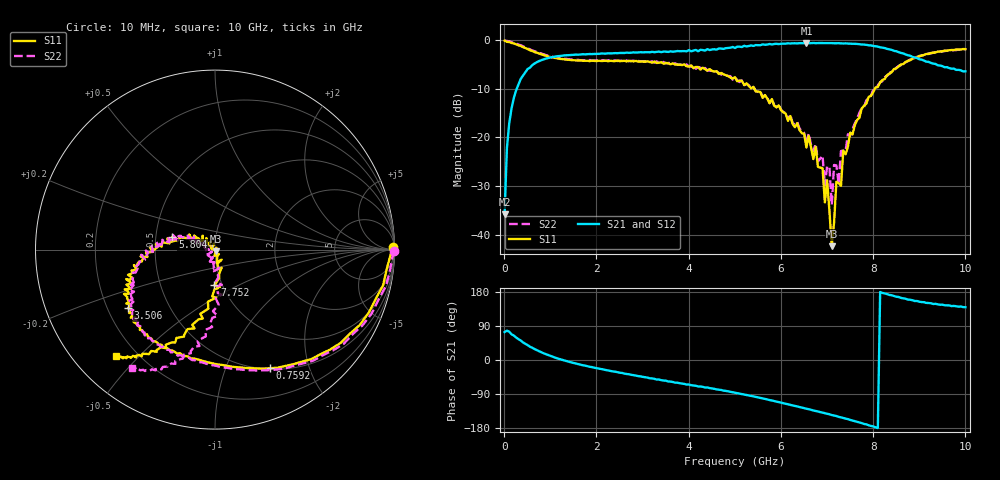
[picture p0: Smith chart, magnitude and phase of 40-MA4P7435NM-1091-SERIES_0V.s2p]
!Agilent Technologies,E8364C,MY48140145,A.09.42.15
!Agilent E8364C: A.09.42.15
!Date: Wednesday, December 02, 2020 13:39:51
!Correction: S11(Full 2 Port(1,2))
!S21(Full 2 Port(1,2))
!S12(Full 2 Port(1,2))
!S22(Full 2 Port(1,2))
!S2P File: Measurements: S11, S21, S12, S22:
# Hz S  dB  R 50
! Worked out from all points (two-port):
!   201 points, 10 MHz to 10 GHz, reference 50 ohm
!   highest |S21| = -0.57 dB at 6.553 GHz (marker M1); lowest = -35.8 dB at 10 MHz (marker M2)
!   |S21| within 3 dB of the highest: 994.4 MHz to 8.913 GHz (7.918 GHz wide, 160 % of centre)
!   lowest |S11| = -42.3 dB at 7.103 GHz (marker M3), VSWR 1.02, Z = 50.3 - j0.713 ohm
!   |S11| at or under -10 dB: 5.427 GHz to 8.037 GHz (2.611 GHz wide, 38.8 % of centre)
!   |S22| runs from -33.9 to 0.0 dB; largest |S21 - S12| = 0.023
!   S11 on the Smith chart (normalised r, x): 10 MHz: open; 759.2 MHz: 0.51, -1.44; 3.506 GHz: 0.29, -0.28; 5.804 GHz: 0.61, +0.09; 7.752 GHz: 0.92, -0.38; 10 GHz: 0.12, -0.43
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1e7  -0.10 0.7  -35.76 73.6  -37.67 50.6  -0.05 -0.4
5.995e7  -0.33 -6.7  -22.20 77.4  -22.18 78.0  -0.16 -6.5
1.5985e8  -0.57 -17.2  -14.07 67.7  -14.10 67.7  -0.42 -17.0
7.5925e8  -2.75 -65.2  -4.28 22.9  -4.28 23.0  -2.61 -65.0
1.7083e9  -4.23 -104.1  -2.88 -13.9  -2.88 -13.5  -4.11 -105.2
3.35665e9  -4.63 -143.0  -2.34 -51.5  -2.36 -52.4  -4.59 -138.1
3.5065e9  -4.67 -146.0  -2.35 -54.5  -2.28 -55.7  -4.76 -140.7
5.005e9  -7.61 -174.8  -1.60 -86.3  -1.54 -85.9  -7.69 -176.0
5.8042e9  -12.10 163.2  -0.88 -106.9  -0.85 -107.0  -12.09 160.8
6.55345e9  -22.06 149.1  -0.57 -128.6  -0.56 -128.2  -21.24 152.7
6.7033e9  -24.43 137.7  -0.57 -133.2  -0.54 -132.8  -22.82 145.9
6.9031e9  -26.32 129.7  -0.60 -138.8  -0.61 -139.1  -23.72 -177.8
6.95305e9  -33.36 160.6  -0.58 -140.4  -0.56 -140.2  -29.80 -179.0
7.003e9  -28.82 98.0  -0.61 -142.0  -0.58 -142.0  -25.86 173.3
7.1029e9  -42.35 -68.4  -0.59 -145.3  -0.57 -144.7  -33.86 -145.8
7.2028e9  -29.12 -95.2  -0.63 -147.9  -0.60 -147.9  -25.75 -106.5
7.25275e9  -29.37 -49.6  -0.61 -150.0  -0.61 -149.7  -29.53 -106.3
7.3027e9  -29.93 -63.9  -0.65 -151.4  -0.65 -151.7  -22.79 -113.2
7.35265e9  -22.72 -81.9  -0.67 -153.0  -0.64 -152.7  -22.71 -81.9
7.75225e9  -14.02 -91.0  -0.88 -166.5  -0.85 -166.4  -13.97 -79.0
8.35165e9  -6.87 -104.6  -1.87 171.7  -1.84 172.5  -6.93 -96.8
1e10  -1.83 -133.0  -6.39 139.3  -6.37 139.2  -1.88 -125.2
